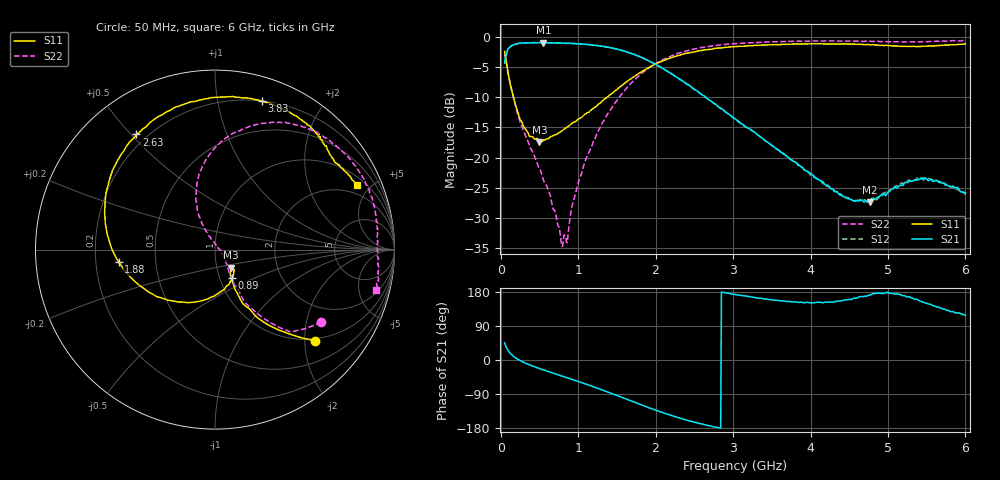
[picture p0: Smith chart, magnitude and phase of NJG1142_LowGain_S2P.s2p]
! Created Thu Jun  3 17:41:04 2010
# hz S ma R 50
! 2 Port Network Data from SP7.SP block
! freq  magS11  angS11  magS21  angS21  magS12  angS12  magS22  angS22
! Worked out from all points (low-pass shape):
!   596 points, 50 MHz to 6 GHz, reference 50 ohm
!   highest |S21| = -0.99 dB at 550 MHz (marker M1); lowest = -27.3 dB at 4.77 GHz (marker M2)
!   |S21| within 3 dB of the highest: 53.46 MHz to 1.907 GHz (1.853 GHz wide, 189 % of centre)
!   lowest |S11| = -17.4 dB at 500 MHz (marker M3), VSWR 1.31, Z = 58.4 - j12 ohm
!   |S11| at or under -10 dB: 164.4 MHz to 1.374 GHz (1.21 GHz wide, 157 % of centre)
!   |S22| runs from -34.6 to -0.6 dB; largest |S21 - S12| = 0.033
!   S11 on the Smith chart (normalised r, x): 50 MHz: 0.95, -2.25; 890 MHz: 1.15, -0.38; 1.88 GHz: 0.30, -0.06; 2.63 GHz: 0.16, +0.52; 3.83 GHz: 0.20, +1.34; 6 GHz: 1.41, +4.16
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5e7  0.7561 -42.2  0.6181 45.6  0.5942 43.5  0.7178 -34.4
1e8  0.4817 -56.4  0.7986 24.0  0.79 23.8  0.4767 -54.3
1.7e8  0.3058 -63.0  0.8565 8.3  0.8632 8.6  0.3041 -60.6
3.1e8  0.1764 -58.8  0.8843 -7.6  0.882 -7.8  0.1571 -58.7
5e8  0.1348 -48.6  0.8918 -22.6  0.8922 -22.5  0.08028 -43.7
5.5e8  0.1391 -46.9  0.8927 -26.1  0.8908 -26.1  0.06579 -40.7
7.9e8  0.1668 -51.1  0.884 -42.2  0.8856 -42.4  0.01858 23.5
8.6e8  0.1797 -55.9  0.8806 -47.0  0.8816 -47.2  0.01984 75.6
8.9e8  0.185 -59.0  0.8809 -49.2  0.8798 -49.3  0.03001 84.7
1.05e9  0.217 -73.8  0.8665 -60.1  0.8674 -60.2  0.07665 112.1
1.28e9  0.2812 -100.1  0.8369 -76.8  0.8386 -76.9  0.1758 115.6
1.53e9  0.38 -131.8  0.779 -96.0  0.7791 -96.4  0.3151 109.9
1.88e9  0.5415 -172.8  0.6449 -123.4  0.6449 -123.6  0.5316 93.3
2.04e9  0.6102 170.9  0.573 -135.3  0.5685 -135.3  0.6181 85.2
2.63e9  0.7773 124.4  0.3235 -170.4  0.3197 -170.6  0.819 58.9
3.03e9  0.8269 102.5  0.2085 172.8  0.2074 172.7  0.8733 45.6
3.83e9  0.8677 72.5  0.08898 152.9  0.08829 153.2  0.916 26.7
4.02e9  0.8701 67.1  0.07294 150.9  0.07174 152.3  0.9206 22.8
4.77e9  0.8531 47.6  0.04297 171.3  0.04447 173.3  0.9156 8.4
5.01e9  0.843 42.5  0.052 176.5  0.05184 176.3  0.9063 4.3
5.48e9  0.8334 34.5  0.06736 151.0  0.06819 150.9  0.9131 -3.2
6e9  0.8693 24.4  0.05156 117.7  0.04915 117.6  0.9263 -14.2
